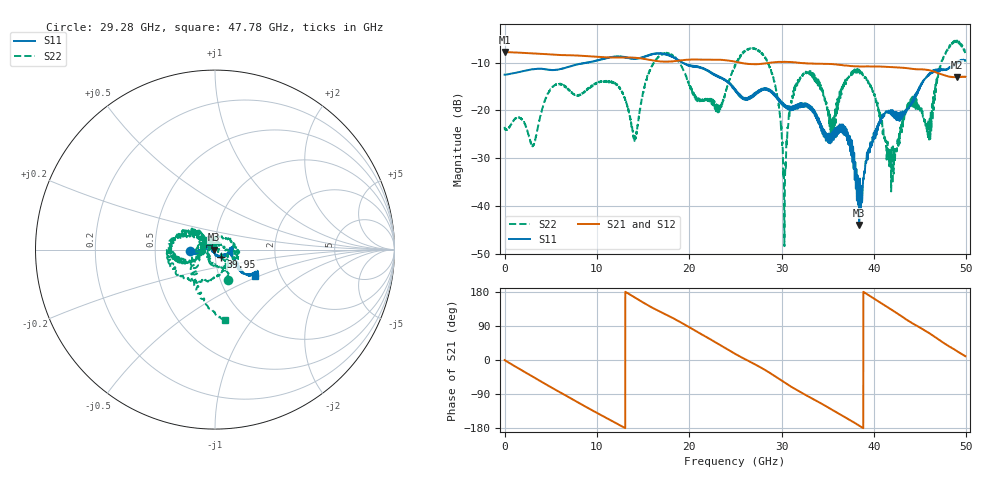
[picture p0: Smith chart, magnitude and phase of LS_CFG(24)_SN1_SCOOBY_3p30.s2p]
!Keysight Technologies,N5245B,MY58422026,A.13.80.08
!Date: Thursday, March 19, 2020 23:34:15
!Correction: S11(Full 2 Port(1,2))
!S21(Full 2 Port(1,2))
!S12(Full 2 Port(1,2))
!S22(Full 2 Port(1,2))
!S2P File: Measurements: S11, S21, S12, S22:
# Hz S DB R 50.0
!freq dBS11 angS11 dBS21 angS21 dBS12 angS12 dBS22 angS22
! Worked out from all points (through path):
!   4991 points, 10 MHz to 49.91 GHz, reference 50 ohm
!   highest |S21| = -7.78 dB at 20 MHz (marker M1); lowest = -13.1 dB at 49.01 GHz (marker M2)
!   group delay of S21, straight-line fit = 39.1 ps
!   lowest |S11| = -44.0 dB at 38.41 GHz (marker M3), VSWR 1.01, Z = 49.4 - j0.0116 ohm
!   |S11| at or under -10 dB: start of sweep to 8.857 GHz; 8.87 GHz to 8.956 GHz (85.54 MHz wide, 0.96 % of centre); 19.24 GHz to 48.88 GHz (29.64 GHz wide, 87 % of centre)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
!   |S22| runs from -48.4 to -5.4 dB; largest |S21 - S12| = 0.0039
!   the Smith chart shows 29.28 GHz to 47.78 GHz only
!   S11 on the Smith chart (normalised r, x): 29.28 GHz: 0.75, -0.01; 39.95 GHz: 1.06, -0.09; 47.78 GHz: 1.48, -0.47
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1e7  -12.53 -1.0  -7.78 -0.2  -7.77 -0.3  -23.46 0.7
2e7  -12.54 -0.6  -7.78 -0.4  -7.77 -0.4  -23.84 -0.9
8.33e9  -10.26 -81.5  -8.58 -117.0  -8.58 -117.0  -16.60 -100.7
1.208e10  -8.73 -108.9  -8.95 -166.7  -8.94 -166.6  -14.42 -91.5
1.412e10  -9.18 -126.3  -8.99 164.9  -8.99 164.9  -26.06 -140.9
1.665e10  -8.09 -137.8  -9.71 129.8  -9.70 129.8  -8.87 -166.5
2.312e10  -13.02 -173.7  -9.40 42.9  -9.40 42.9  -20.40 -149.3
2.496e10  -15.63 -176.5  -9.79 16.4  -9.78 16.5  -10.72 -168.4
2.928e10  -17.00 -177.2  -9.91 -42.6  -9.91 -42.5  -14.76 -66.2
3.028e10  -18.72 -173.4  -9.85 -58.6  -9.85 -58.5  -38.12 27.3
3.128e10  -19.37 -167.1  -9.94 -74.0  -9.93 -73.9  -15.91 149.5
3.328e10  -19.54 -176.1  -10.21 -101.4  -10.21 -101.1  -12.28 -170.8
3.552e10  -26.01 150.0  -10.32 -131.9  -10.25 -131.5  -25.11 174.4
3.714e10  -24.54 142.0  -10.66 -154.8  -10.56 -154.9  -13.39 154.6
3.841e10  -44.01 -178.9  -10.82 -173.3  -10.77 -173.6  -11.49 -157.5
3.995e10  -25.29 -52.6  -10.80 163.0  -10.77 162.8  -16.06 -88.9
4.16e10  -20.17 5.3  -10.92 137.5  -10.94 137.4  -28.69 88.6
4.4e10  -18.76 -24.9  -11.26 99.4  -11.27 99.4  -17.68 -35.0
4.6e10  -12.60 -37.1  -11.62 70.6  -11.64 70.6  -24.63 123.2
4.778e10  -11.49 -33.6  -12.72 41.4  -12.72 41.4  -8.03 -82.0
4.901e10  -9.82 -47.6  -13.06 23.2  -13.08 23.2  -5.37 -43.5
4.991e10  -9.60 -43.3  -12.96 9.9  -12.98 9.8  -8.03 -16.0
